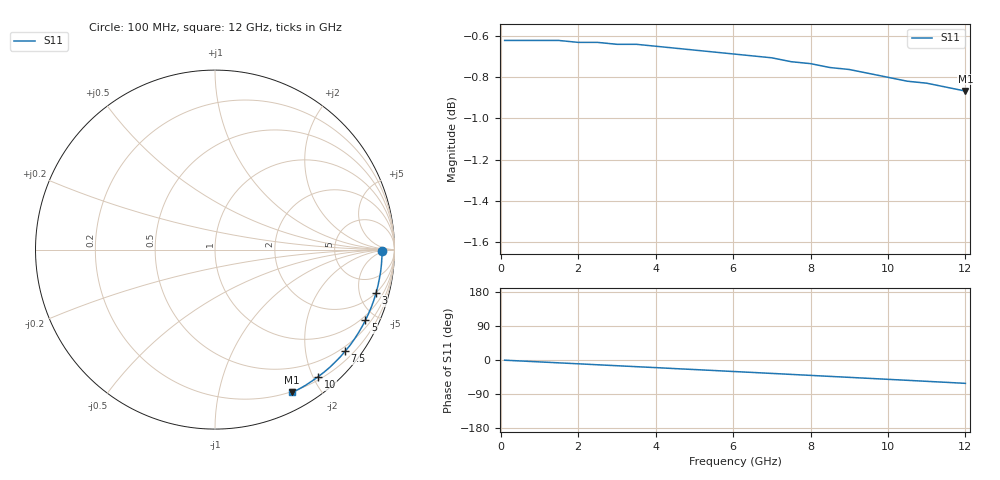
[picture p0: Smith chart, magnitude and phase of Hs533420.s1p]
!HSCH-5314 and HSCH-5334 Schottky diodes
!S-parameters at 20 microamp external bias.  Last updated 6/7/94
# ghz s ma r 50
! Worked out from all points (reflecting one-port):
!   25 points, 100 MHz to 12 GHz, reference 50 ohm
!   lowest |S11| = -0.9 dB at 12 GHz (marker M1), VSWR 20.05, Z = 9.44 - j83.1 ohm
!   phase of S11 starts at -0 deg and turns -61 deg over the sweep
!   S11 on the Smith chart (normalised r, x): 100 MHz: 28, -3; 3 GHz: 1.98, -7.00; 5 GHz: 0.78, -4.34; 7.5 GHz: 0.39, -2.86; 10 GHz: 0.25, -2.07; 12 GHz: 0.19, -1.66
0.1  0.931 -0.5
0.5  0.931 -2.5
1  0.931 -5.0
1.5  0.931 -7.5
2  0.93 -10.0
2.5  0.93 -12.6
3  0.929 -15.1
3.5  0.929 -17.6
4  0.928 -20.1
4.5  0.927 -22.7
5  0.926 -25.2
5.5  0.925 -27.7
6  0.924 -30.3
6.5  0.923 -32.8
7  0.922 -35.4
7.5  0.92 -38.0
8  0.919 -40.6
8.5  0.917 -43.2
9  0.916 -45.8
9.5  0.914 -48.4
10  0.912 -51.0
10.5  0.91 -53.6
11  0.909 -56.3
11.5  0.907 -58.9
12  0.905 -61.6
